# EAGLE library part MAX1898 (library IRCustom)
Maxim MAX1898 li-poly battery charger http://www.ladyada.net/library/eagle
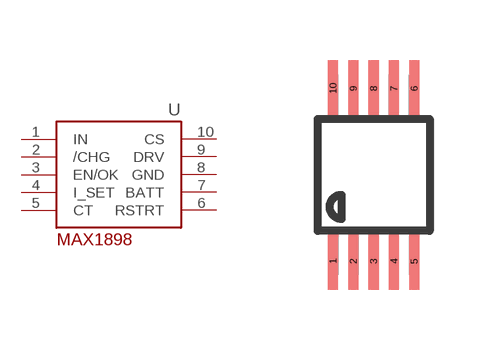
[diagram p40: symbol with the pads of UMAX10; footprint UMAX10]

Designator prefix -

## MAX1898U  [UMAX10]
1  IN  in
2  /CHG  out
3  EN/OK  in
4  I_SET  pas
5  CT  pas
6  RSTRT  pas
7  BATT  out
8  GND  pwr
9  DRV  out
10  CS  in

## Footprint UMAX10 (pad centres in mm)
smd 0.254 x 1.422: 1 -1.016,-2.159; 2 -0.508,-2.159; 3 0,-2.159; 4 0.508,-2.159; 5 1.016,-2.159; 6 1.016,2.159; 7 0.508,2.159; 8 0,2.159; 9 -0.508,2.159; 10 -1.016,2.159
